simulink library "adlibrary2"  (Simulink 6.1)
undefined symbols (not defined in the file or in its folder): adlibrary2, ADM, Bit, Black, Box, d2sram_config, DDR, ddr32_config, ddr32xp_config, Generation, II, Inactive, Location, Lower, SDRAM, Simulation, Subsystem, Width, xbsIndex_r3, XPL, XRC, XRM, zbt32_config, zbt64_config, zbtXRC4_config
libraries: xbsIndex_r3 x786
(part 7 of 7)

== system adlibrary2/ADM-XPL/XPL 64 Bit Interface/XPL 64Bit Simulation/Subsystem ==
  data_write0 : Inport  Port=1  LatchInput=off
  data_write1 : Inport  Port=2  LatchInput=off
  addr : Inport  Port=3  LatchInput=off
  be : Inport  Port=4  LatchInput=off
  write : Inport  Port=5  LatchInput=off
  read : Inport  Port=6  LatchInput=off
  control0 : Inport  Port=7  LatchInput=off
  control1 : Inport  Port=8  LatchInput=off
  ififo_data0 : Inport  Port=9  LatchInput=off
  ififo_data1 : Inport  Port=10  LatchInput=off
  ififo_empty : Inport  Port=11  LatchInput=off
  ofifo_full : Inport  Port=12  LatchInput=off
  Concat : xbsIndex_r3/Concat  num_inputs=2  explicit_period=off  period=1  dbl_ovrd=off
  Concat1 : xbsIndex_r3/Concat  num_inputs=2  explicit_period=off  period=1  dbl_ovrd=off
  Concat2 : xbsIndex_r3/Concat  num_inputs=2  explicit_period=off  period=1  dbl_ovrd=off
  Disregard Subsystem : xbsIndex_r3/Disregard Subsystem  Tag=discardX
  Gateway In{,1..2,6..7,9} (6 alike) : xbsIndex_r3/Gateway In  arith_type=Unsigned  n_bits=32  bin_pt=0  quantization=Truncate  overflow=Wrap  period=1  timing_constraint=None  locs_specified=off  LOCs={}  needs_fixed_name=off  dbl_ovrd=off  show_param=off
  Gateway In10 : xbsIndex_r3/Gateway In  arith_type=Boolean  n_bits=8  bin_pt=6  quantization=Truncate  overflow=Wrap  period=1  timing_constraint=None  locs_specified=off  LOCs={}  needs_fixed_name=off  dbl_ovrd=off  show_param=off
  Gateway In11 : xbsIndex_r3/Gateway In  arith_type=Boolean  n_bits=8  bin_pt=6  quantization=Truncate  overflow=Wrap  period=1  timing_constraint=None  locs_specified=off  LOCs={}  needs_fixed_name=off  dbl_ovrd=off  show_param=off
  Gateway In3 : xbsIndex_r3/Gateway In  arith_type=Boolean  n_bits=32  bin_pt=0  quantization=Truncate  overflow=Wrap  period=1  timing_constraint=None  locs_specified=off  LOCs={}  needs_fixed_name=off  dbl_ovrd=off  show_param=off
  Gateway In4 : xbsIndex_r3/Gateway In  arith_type=Boolean  n_bits=8  bin_pt=6  quantization=Truncate  overflow=Wrap  period=1  timing_constraint=None  locs_specified=off  LOCs={}  needs_fixed_name=off  dbl_ovrd=off  show_param=off
  Gateway In5 : xbsIndex_r3/Gateway In  arith_type=Unsigned  n_bits=8  bin_pt=0  quantization=Truncate  overflow=Wrap  period=1  timing_constraint=None  locs_specified=off  LOCs={}  needs_fixed_name=off  dbl_ovrd=off  show_param=off
  Gateway In8 : xbsIndex_r3/Gateway In  arith_type=Unsigned  n_bits=16  bin_pt=0  quantization=Truncate  overflow=Wrap  period=1  timing_constraint=None  locs_specified=off  LOCs={}  needs_fixed_name=off  dbl_ovrd=off  show_param=off
  Out1 : Outport
  Out2 : Outport  Port=2
  Out3 : Outport  Port=3
  Out4 : Outport  Port=4
  Out5 : Outport  Port=5
  Out6 : Outport  Port=6
  Out7 : Outport  Port=7
  Out8 : Outport  Port=8
  Out9 : Outport  Port=9
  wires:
  data_write0/1 -> Gateway In7/1
  data_write1/1 -> Gateway In6/1
  be/1 -> Gateway In5/1
  write/1 -> Gateway In4/1
  read/1 -> Gateway In3/1
  control0/1 -> Gateway In2/1
  control1/1 -> Gateway In1/1
  ififo_data0/1 -> Gateway In/1
  addr/1 -> Gateway In8/1
  Gateway In6/1 -> Concat/1
  Gateway In7/1 -> Concat/2
  Concat/1 -> Out1/1
  Gateway In8/1 -> Out2/1
  Gateway In5/1 -> Out3/1
  Gateway In4/1 -> Out4/1
  Gateway In3/1 -> Out5/1
  Gateway In2/1 -> Concat1/2
  Gateway In1/1 -> Concat1/1
  Concat1/1 -> Out6/1
  ififo_data1/1 -> Gateway In9/1
  ififo_empty/1 -> Gateway In10/1
  ofifo_full/1 -> Gateway In11/1
  Gateway In9/1 -> Concat2/1
  Gateway In/1 -> Concat2/2
  Concat2/1 -> Out7/1
  Gateway In10/1 -> Out8/1
  Gateway In11/1 -> Out9/1

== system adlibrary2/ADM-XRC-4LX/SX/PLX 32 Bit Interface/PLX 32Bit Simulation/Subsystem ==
  In1 : Inport  Port=1  LatchInput=off
  In2 : Inport  Port=2  LatchInput=off
  In9 : Inport  Port=3  LatchInput=off
  In3 : Inport  Port=4  LatchInput=off
  In4 : Inport  Port=5  LatchInput=off
  In5 : Inport  Port=6  LatchInput=off
  In6 : Inport  Port=7  LatchInput=off
  In7 : Inport  Port=8  LatchInput=off
  In8 : Inport  Port=9  LatchInput=off
  Disregard Subsystem : xbsIndex_r3/Disregard Subsystem  Tag=discardX
  Gateway In{,1,4..5} (4 alike) : xbsIndex_r3/Gateway In  arith_type=Boolean  n_bits=8  bin_pt=6  quantization=Truncate  overflow=Wrap  period=1  timing_constraint=None  locs_specified=off  LOCs={}  needs_fixed_name=off  dbl_ovrd=off  show_param=off
  Gateway In2 : xbsIndex_r3/Gateway In  arith_type=Unsigned  n_bits=32  bin_pt=0  quantization=Truncate  overflow=Wrap  period=1  timing_constraint=None  locs_specified=off  LOCs={}  needs_fixed_name=off  dbl_ovrd=off  show_param=off
  Gateway In3 : xbsIndex_r3/Gateway In  arith_type=Unsigned  n_bits=32  bin_pt=0  quantization=Truncate  overflow=Wrap  period=1  timing_constraint=None  locs_specified=off  LOCs={}  needs_fixed_name=off  dbl_ovrd=off  show_param=off
  Gateway In6 : xbsIndex_r3/Gateway In  arith_type=Unsigned  n_bits=16  bin_pt=0  quantization=Truncate  overflow=Wrap  period=1  timing_constraint=None  locs_specified=off  LOCs={}  needs_fixed_name=off  dbl_ovrd=off  show_param=off
  Gateway In7 : xbsIndex_r3/Gateway In  arith_type=Unsigned  n_bits=32  bin_pt=0  quantization=Truncate  overflow=Wrap  period=1  timing_constraint=None  locs_specified=off  LOCs={}  needs_fixed_name=off  dbl_ovrd=off  show_param=off
  Gateway In8 : xbsIndex_r3/Gateway In  arith_type=Unsigned  n_bits=4  bin_pt=0  quantization=Truncate  overflow=Wrap  period=1  timing_constraint=None  locs_specified=off  LOCs={}  needs_fixed_name=off  dbl_ovrd=off  show_param=off
  Out1 : Outport
  Out2 : Outport  Port=2
  Out9 : Outport  Port=3
  Out3 : Outport  Port=4
  Out4 : Outport  Port=5
  Out5 : Outport  Port=6
  Out6 : Outport  Port=7
  Out7 : Outport  Port=8
  Out8 : Outport  Port=9
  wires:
  Gateway In8/1 -> Out9/1
  In9/1 -> Gateway In8/1
  Gateway In7/1 -> Out1/1
  Gateway In6/1 -> Out2/1
  Gateway In5/1 -> Out3/1
  Gateway In4/1 -> Out4/1
  Gateway In3/1 -> Out5/1
  Gateway In2/1 -> Out6/1
  Gateway In1/1 -> Out7/1
  Gateway In/1 -> Out8/1
  In8/1 -> Gateway In/1
  In7/1 -> Gateway In1/1
  In6/1 -> Gateway In2/1
  In5/1 -> Gateway In3/1
  In4/1 -> Gateway In4/1
  In3/1 -> Gateway In5/1
  In2/1 -> Gateway In6/1
  In1/1 -> Gateway In7/1

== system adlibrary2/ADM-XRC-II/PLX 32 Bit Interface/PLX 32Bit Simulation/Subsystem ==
  In1 : Inport  Port=1  LatchInput=off
  In2 : Inport  Port=2  LatchInput=off
  In9 : Inport  Port=3  LatchInput=off
  In3 : Inport  Port=4  LatchInput=off
  In4 : Inport  Port=5  LatchInput=off
  In5 : Inport  Port=6  LatchInput=off
  In6 : Inport  Port=7  LatchInput=off
  In7 : Inport  Port=8  LatchInput=off
  In8 : Inport  Port=9  LatchInput=off
  Disregard Subsystem : xbsIndex_r3/Disregard Subsystem  Tag=discardX
  Gateway In{,1,4..5} (4 alike) : xbsIndex_r3/Gateway In  arith_type=Boolean  n_bits=8  bin_pt=6  quantization=Truncate  overflow=Wrap  period=1  timing_constraint=None  locs_specified=off  LOCs={}  needs_fixed_name=off  dbl_ovrd=off  show_param=off
  Gateway In2 : xbsIndex_r3/Gateway In  arith_type=Unsigned  n_bits=32  bin_pt=0  quantization=Truncate  overflow=Wrap  period=1  timing_constraint=None  locs_specified=off  LOCs={}  needs_fixed_name=off  dbl_ovrd=off  show_param=off
  Gateway In3 : xbsIndex_r3/Gateway In  arith_type=Unsigned  n_bits=32  bin_pt=0  quantization=Truncate  overflow=Wrap  period=1  timing_constraint=None  locs_specified=off  LOCs={}  needs_fixed_name=off  dbl_ovrd=off  show_param=off
  Gateway In6 : xbsIndex_r3/Gateway In  arith_type=Unsigned  n_bits=16  bin_pt=0  quantization=Truncate  overflow=Wrap  period=1  timing_constraint=None  locs_specified=off  LOCs={}  needs_fixed_name=off  dbl_ovrd=off  show_param=off
  Gateway In7 : xbsIndex_r3/Gateway In  arith_type=Unsigned  n_bits=32  bin_pt=0  quantization=Truncate  overflow=Wrap  period=1  timing_constraint=None  locs_specified=off  LOCs={}  needs_fixed_name=off  dbl_ovrd=off  show_param=off
  Gateway In8 : xbsIndex_r3/Gateway In  arith_type=Unsigned  n_bits=4  bin_pt=0  quantization=Truncate  overflow=Wrap  period=1  timing_constraint=None  locs_specified=off  LOCs={}  needs_fixed_name=off  dbl_ovrd=off  show_param=off
  Out1 : Outport
  Out2 : Outport  Port=2
  Out9 : Outport  Port=3
  Out3 : Outport  Port=4
  Out4 : Outport  Port=5
  Out5 : Outport  Port=6
  Out6 : Outport  Port=7
  Out7 : Outport  Port=8
  Out8 : Outport  Port=9
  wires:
  Gateway In8/1 -> Out9/1
  In9/1 -> Gateway In8/1
  Gateway In7/1 -> Out1/1
  Gateway In6/1 -> Out2/1
  Gateway In5/1 -> Out3/1
  Gateway In4/1 -> Out4/1
  Gateway In3/1 -> Out5/1
  Gateway In2/1 -> Out6/1
  Gateway In1/1 -> Out7/1
  Gateway In/1 -> Out8/1
  In8/1 -> Gateway In/1
  In7/1 -> Gateway In1/1
  In6/1 -> Gateway In2/1
  In5/1 -> Gateway In3/1
  In4/1 -> Gateway In4/1
  In3/1 -> Gateway In5/1
  In2/1 -> Gateway In6/1
  In1/1 -> Gateway In7/1

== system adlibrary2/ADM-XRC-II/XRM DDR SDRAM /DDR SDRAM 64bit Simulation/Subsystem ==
  In1 : Inport  Port=1  LatchInput=off
  In2 : Inport  Port=2  LatchInput=off
  In3 : Inport  Port=3  LatchInput=off
  Disregard Subsystem : xbsIndex_r3/Disregard Subsystem  Tag=discardX
  g02 : xbsIndex_r3/Gateway In  arith_type=Unsigned  n_bits=3  bin_pt=0  quantization=Truncate  overflow=Wrap  period=1  timing_constraint=None  locs_specified=off  LOCs={}  needs_fixed_name=off  dbl_ovrd=off  show_param=off
  go0 : xbsIndex_r3/Gateway In  arith_type=Unsigned  n_bits=32  bin_pt=0  quantization=Truncate  overflow=Wrap  period=1  timing_constraint=None  locs_specified=off  LOCs={}  needs_fixed_name=off  dbl_ovrd=off  show_param=off
  go1 : xbsIndex_r3/Gateway In  arith_type=Boolean  n_bits=32  bin_pt=0  quantization=Truncate  overflow=Wrap  period=1  timing_constraint=None  locs_specified=off  LOCs={}  needs_fixed_name=off  dbl_ovrd=off  show_param=off
  Out1 : Outport
  Out2 : Outport  Port=2
  Out3 : Outport  Port=3
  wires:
  In1/1 -> go0/1
  In2/1 -> go1/1
  In3/1 -> g02/1
  go0/1 -> Out1/1
  go1/1 -> Out2/1
  g02/1 -> Out3/1
